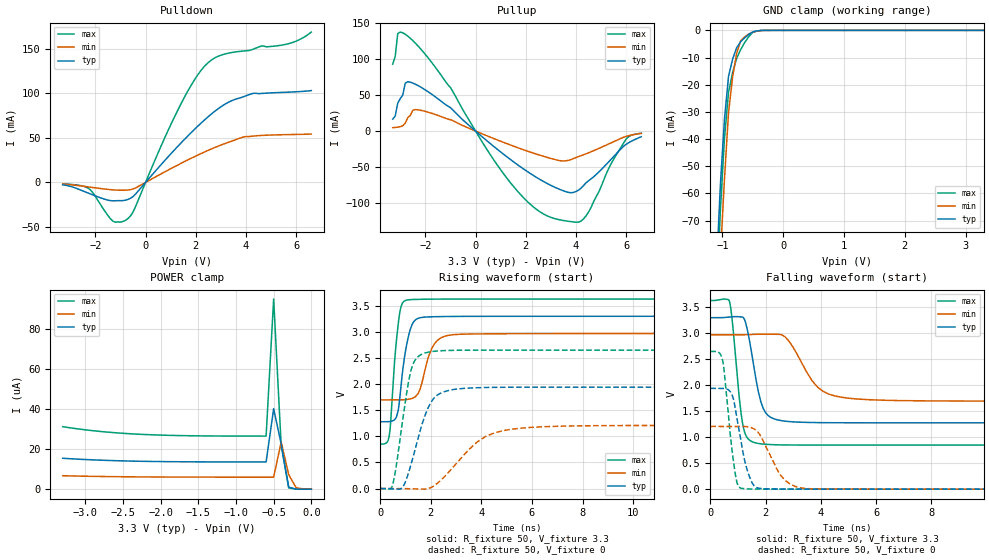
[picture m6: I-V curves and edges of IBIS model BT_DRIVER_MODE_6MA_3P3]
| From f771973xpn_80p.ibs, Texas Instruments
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|   Model Cell BT_DRIVER_MODE_6MA_3P3
|BT_DRIVER_MODE_6MA_3P3
[Model]   BT_DRIVER_MODE_6MA_3P3
Model_type   I/O
Polarity   Non-Inverting
Enable   Active-Low
Vinl =  0.8
Vinh =  2
Cref =  15.0000pF
Rref =  100.0000M
Vref =  0V
Vmeas =  1.65
C_comp   3.98845p   2.03906p   4.55356p
[Model Spec]
Vinl   0.8   0.8   0.8
Vinh   2   2   2
[Temperature Range]   25   155   -40
[Voltage Range]   3.3   2.97   3.63
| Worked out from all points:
|   slope of the pulldown table from 0 to 0.495 V, typ, clamps not added: 30.9 ohm
|   slope of the pullup table from 0 to 0.495 V, typ, clamps not added: 33.7 ohm
|   GND clamp passes 1 mA (typ) near -0.53 V on its own axis
|   rising waveform, R_fixture 50, V_fixture 3.3: 20-80 % time 345ps typ, 467ps min, 263ps max; typ from 1.28 V to 3.3 V
|   rising waveform, R_fixture 50, V_fixture 0: 20-80 % time 724ps typ, 1.5ns min, 484ps max; typ from 0 V to 1.94 V
|   falling waveform, R_fixture 50, V_fixture 3.3: 20-80 % time 422ps typ, 899ps min, 301ps max; typ from 3.3 V to 1.28 V
|   falling waveform, R_fixture 50, V_fixture 0: 20-80 % time 420ps typ, 709ps min, 309ps max; typ from 1.94 V to 0 V
| Nom Voltages:
|   BIASFET=3.3, VDD=1.2, VDDS=3.3, VSS=0
| Min Voltages:
|   BIASFET=2.97, VDD=1.08, VDDS=2.97, VSS=0
| Max Voltages:
|   BIASFET=3.63, VDD=1.32, VDDS=3.63, VSS=0
[POWER_clamp]
|   voltage   I(typ)   I(min)   I(max)
-3.3V     15.41uA    6.707uA    31.17uA
-2.8V     14.47uA    6.332uA    28.78uA
-2.2V     13.87uA    6.102uA    27.25uA
-1.6V     13.64uA    6.016uA    26.64uA
-600mV    13.58uA    5.99uA     26.46uA
-500mV    40.13uA    5.991uA    94.83uA
-400mV    22.54uA    23.52uA    21.76uA
-300mV    969.1nA    7.216uA    616.4nA
-200mV    29.93nA    661.1nA    11.88nA
0V        1.388nA    48.32nA    1.243nA
[Pulldown]
|   voltage   I(typ)   I(min)   I(max)
-3.3V     -2.737mA   -1.873mA   -1.718mA
-2.3V     -11.76mA   -4.954mA   -6.193mA
-1.3V     -20.63mA   -8.362mA   -43.49mA
-800mV    -19.88mA   -8.768mA   -42.58mA
-500mV    -15.9mA    -7.318mA   -33.21mA
1.4V      43.88mA    21.19mA    87.52mA
1.9V      58.17mA    28.19mA    112.9mA
2.4V      71.33mA    34.76mA    131.7mA
3V        84.76mA    41.87mA    142.6mA
4.3V      99.91mA    51.98mA    149.5mA
5.8V      101.3mA    53.65mA    156.4mA
6.6V      102.9mA    54.17mA    168.5mA
[Pullup]
|   voltage   I(typ)   I(min)   I(max)
-3.3V     16.59mA    4.724mA    92.73mA
-3.2V     20.85mA    5.035mA    103.7mA
-3.1V     38.73mA    5.465mA    135.1mA
-2.8V     66.51mA    11.16mA    134.3mA
-2.5V     66.63mA    28.85mA    125.5mA
-1V       32.41mA    15.86mA    60.36mA
1.4V      -39.76mA   -19.48mA   -72.15mA
3.2V      -78.67mA   -39.79mA   -121.9mA
3.8V      -85.6mA    -39.58mA   -125.6mA
4.3V      -75.56mA   -32.88mA   -121.7mA
6V        -18.27mA   -7.323mA   -10.91mA
6.6V      -7.8mA     -3.26mA    -3.094mA
[GND_clamp]
|   voltage   I(typ)   I(min)   I(max)
-3.3V     -1.746A    -1.481A    -2.454A
-1.1V     -88.72mA   -114.8mA   -101.4mA
-1.033V   -56.66mA   -82.94mA   -65.99mA
-966.7mV  -32.75mA   -54.79mA   -39.79mA
-900mV    -16.98mA   -30.37mA   -22.81mA
-833.3mV  -10.67mA   -17.32mA   -15.58mA
-766.7mV  -6.402mA   -8.477mA   -10.34mA
-700mV    -4.171mA   -3.846mA   -7.085mA
-566.7mV  -1.511mA   -1.331mA   -2.329mA
-500mV    -537.7uA   -639.3uA   -683uA
-300mV    -1.439uA   -12.56uA   -707.1nA
3.3V      1.388nA    14.18uA    1.029nA
[Ramp]
| variable   typ   min   max
dV/dt_f  1.2265162/0.42596978n 0.77333606/0.9075597n  1.6862307/0.30383977n
dV/dt_r  1.1726677/0.72864722n 0.73282855/1.5166001n  1.5979937/0.48603734n
R_load = 50
[Rising Waveform]
R_fixture = 50
V_fixture = 3.3
V_fixture_min = 2.97
V_fixture_max = 3.63
|   time   V(typ)   V(min)   V(max)
0s        1.279V     1.698V     849.6mV
345.1ps   1.281V     1.698V     978.7mV
635.1ps   1.364V     1.698V     2.818V
807ps     1.906V     1.698V     3.458V
1.046ns   2.76V      1.705V     3.61V
1.258ns   3.141V     1.726V     3.621V
1.47ns    3.256V     1.806V     3.624V
2.083ns   3.291V     2.727V     3.629V
2.855ns   3.297V     2.946V     3.63V
20.09ns   3.3V       2.97V      3.63V
[Rising Waveform]
R_fixture = 50
V_fixture = 0
V_fixture_min = 0
V_fixture_max = 0
|   time   V(typ)   V(min)   V(max)
0s        0V         0V         0V
471.2ps   -6.127mV   0V         41.96mV
927.4ps   57.41mV    0V         1.45V
1.241ns   504.4mV    -5.315mV   2.309V
1.752ns   1.372V     -12.2mV    2.594V
2.094ns   1.716V     43.23mV    2.628V
2.521ns   1.854V     219.2mV    2.643V
3.834ns   1.932V     892.4mV    2.651V
5.162ns   1.941V     1.134V     2.651V
20.01ns   1.941V     1.208V     2.651V
[Falling Waveform]
R_fixture = 50
V_fixture = 3.3
V_fixture_min = 2.97
V_fixture_max = 3.63
|   time   V(typ)   V(min)   V(max)
0s        3.3V       2.97V      3.63V
685.1ps   3.313V     2.97V      3.627V
1.166ns   3.314V     2.971V     1.274V
1.615ns   2.234V     2.98V      893.3mV
1.83ns    1.68V      2.984V     872mV
2.187ns   1.383V     2.982V     857.8mV
2.8ns     1.303V     2.878V     850.5mV
3.881ns   1.281V     1.963V     848.6mV
4.946ns   1.278V     1.754V     848.5mV
20.09ns   1.279V     1.697V     849mV
[Falling Waveform]
R_fixture = 50
V_fixture = 0
V_fixture_min = 0
V_fixture_max = 0
|   time   V(typ)   V(min)   V(max)
0s        1.94V      1.207V     2.651V
448ps     1.941V     1.207V     2.476V
720.3ps   1.878V     1.207V     1.065V
885.2ps   1.613V     1.207V     358.3mV
1.113ns   921.7mV    1.208V     17.5mV
1.312ns   408.6mV    1.204V     5.492mV
1.591ns   61.74mV    1.158V     2.02mV
2.552ns   2.098mV    262.7mV    0V
3.461ns   0V         11.91mV    0V
20.01ns   0V         0V         0V
